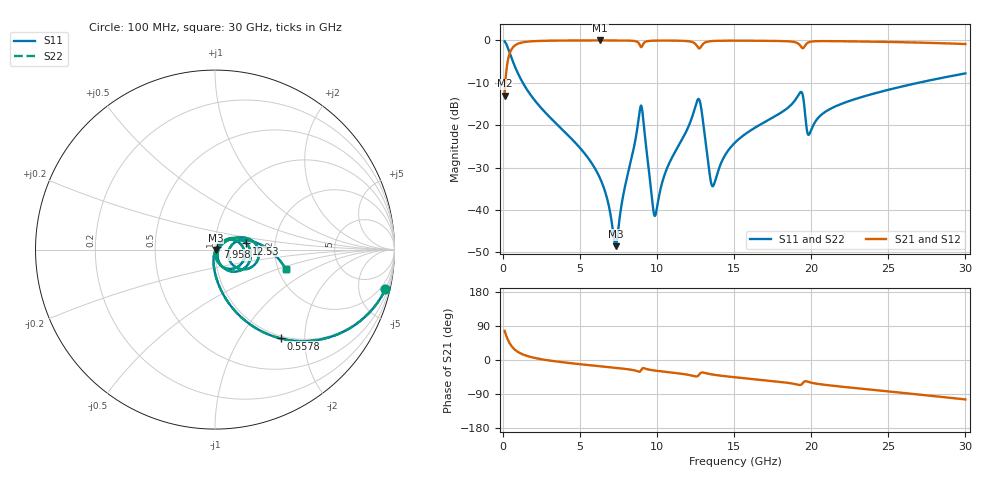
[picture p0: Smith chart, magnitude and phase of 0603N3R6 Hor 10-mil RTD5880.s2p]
# GHz S MA R 50
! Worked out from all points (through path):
!   3201 points, 100 MHz to 30 GHz, reference 50 ohm
!   highest |S21| = -0.03 dB at 6.304 GHz (marker M1); lowest = -13.0 dB at 100 MHz (marker M2)
!   group delay of S21, straight-line fit = 10.8 ps
!   lowest |S11| = -48.5 dB at 7.304 GHz (marker M3), VSWR 1.01, Z = 50.3 - j0.142 ohm
!   |S11| at or under -10 dB: 1.28 GHz to 26.96 GHz (25.68 GHz wide, 182 % of centre)
!   |S22| runs from -48.5 to -0.2 dB; largest |S21 - S12| = 0
!   S11 on the Smith chart (normalised r, x): 100 MHz: 0.96, -8.56; 557.8 MHz: 0.96, -1.53; 7.958 GHz: 1.03, +0.03; 12.53 GHz: 1.42, +0.10; 30 GHz: 2.20, -0.56
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0.1  0.9748 -13.2  0.223 76.8  0.223 76.8  0.9748 -13.2
0.5578437  0.6149 -53.6  0.7879 36.4  0.7879 36.4  0.6149 -53.6
0.959625  0.4099 -68.4  0.9112 21.5  0.9112 21.5  0.4099 -68.4
1.613687  0.2523 -79.7  0.9663 10.0  0.9663 10.0  0.2523 -79.7
5.089563  0.0514 -98.8  0.9961 -11.5  0.9961 -11.5  0.0514 -98.8
6.30425  0.02336 -99.3  0.9967 -16.6  0.9967 -16.6  0.02336 -99.3
7.304031  0.00374 -22.2  0.9962 -20.7  0.9962 -20.7  0.00374 -22.2
7.958094  0.02072 50.8  0.9942 -23.7  0.9942 -23.7  0.02072 50.8
8.948531  0.1701 -15.1  0.833 -27.4  0.833 -27.4  0.1701 -15.1
9.752094  0.009938 -47.9  0.9906 -27.3  0.9906 -27.3  0.009938 -47.9
10.06978  0.01301 27.7  0.9927 -29.0  0.9927 -29.0  0.01301 27.7
10.60238  0.02985 46.1  0.993 -31.5  0.993 -31.5  0.02985 46.1
12.52719  0.1786 11.1  0.8859 -43.5  0.8859 -43.5  0.1786 11.1
12.82619  0.1714 -45.4  0.8312 -34.0  0.8312 -34.0  0.1714 -45.4
13.59238  0.01902 -19.2  0.9818 -38.4  0.9818 -38.4  0.01902 -19.2
15.05  0.06224 37.7  0.9906 -45.5  0.9906 -45.5  0.06224 37.7
19.29206  0.2445 -2.8  0.8648 -65.8  0.8648 -65.8  0.2445 -2.8
19.77794  0.07825 -17.7  0.9382 -57.3  0.9382 -57.3  0.07825 -17.7
20.03956  0.09183 12.7  0.9689 -60.2  0.9689 -60.2  0.09183 12.7
21.31966  0.1585 19.3  0.9784 -67.6  0.9784 -67.6  0.1585 19.3
25.01978  0.2616 5.4  0.9576 -83.0  0.9576 -83.0  0.2616 5.4
30  0.4077 -15.2  0.9045 -104.1  0.9045 -104.1  0.4077 -15.2
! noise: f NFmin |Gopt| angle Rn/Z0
0.1  0.0003755  0.9372  0.8227  0.001334
3.417  0.003836  0.8011  9.875  0.003969
6.743  0.006862  0.7837  19.15  0.006338
10.06  0.0125  0.8207  28.36  0.01374
13.39  0.02747  0.8885  37.5  0.04807
16.7  0.01549  0.7715  46.21  0.01173
20.03  0.03428  0.871  55.09  0.04504
23.35  0.01899  0.7499  63.09  0.01119
26.67  0.02087  0.7447  71.1  0.01099
30  0.02341  0.7475  78.89  0.01128
